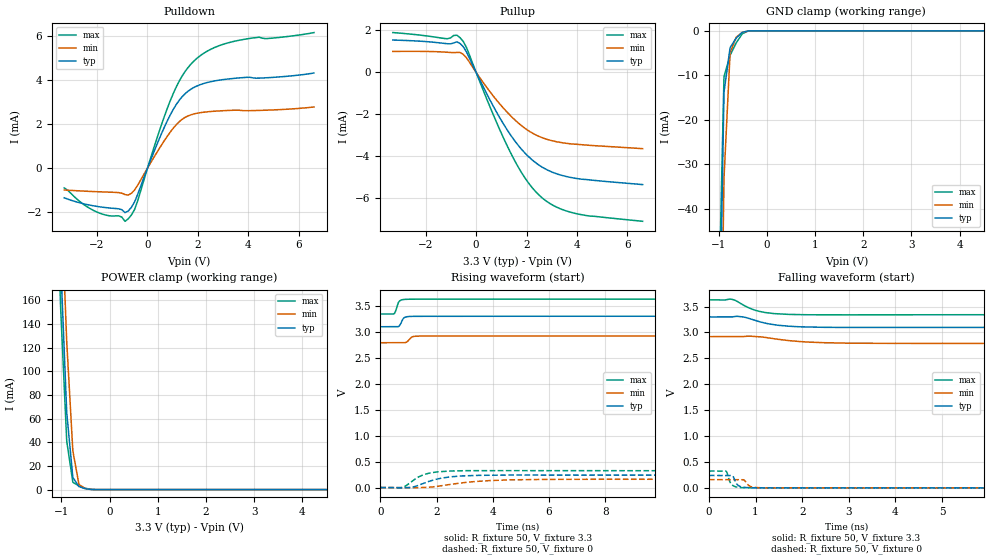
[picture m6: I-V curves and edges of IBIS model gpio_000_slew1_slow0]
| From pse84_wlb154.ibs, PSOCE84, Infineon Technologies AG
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[Model] gpio_000_slew1_slow0
Model_type I/O
Enable   Active-High
Vinl  =  0.99
Vinh  =  2.31
Vmeas =  1.65
Cref  =  15e-12
| Capacitance   typ   min   max
C_comp   1.09946e-12   1.086232e-12   1.114407e-12
| Variables   typ   min   max
[GND Clamp Reference]   0   0   0
[POWER Clamp Reference]   3.3   2.92   3.63
[Pulldown Reference]   0   0   0
[Pullup Reference]   3.3   2.92   3.63
[Temperature Range]   25   125   -40
[Voltage Range]   3.3   2.92   3.63
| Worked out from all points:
|   slope of the pulldown table from 0 to 0.495 V, typ, clamps not added: 352 ohm
|   slope of the pullup table from 0 to 0.495 V, typ, clamps not added: 415 ohm
|   GND clamp passes 1 mA (typ) near -0.57 V on its own axis
|   POWER clamp passes 1 mA (typ) near -0.52 V on its own axis
|   falling waveform, R_fixture 50, V_fixture 3.3: 20-80 % time 594ps typ, 820ps min, 464ps max; typ from 3.3 V to 3.1 V
|   falling waveform, R_fixture 50, V_fixture 0: 20-80 % time 91.4ps typ, 98.1ps min, 88.6ps max; typ from 0.239 V to 0 V
|   rising waveform, R_fixture 50, V_fixture 3.3: 20-80 % time 118ps typ, 140ps min, 107ps max; typ from 3.1 V to 3.3 V
|   rising waveform, R_fixture 50, V_fixture 0: 20-80 % time 912ps typ, 1.55ns min, 627ps max; typ from 0 V to 0.239 V
[GND Clamp]
| Voltage   I(typ)   I(min)   I(max)
-1.65V    -892.5mA   -911.9mA   -883.9mA
-1.015V   -92.32mA   -129.7mA   -71.28mA
-888.3mV  -13.83mA   -33.21mA   -10.31mA
-761.4mV  -3.792mA   -4.944mA   -5.509mA
-634.5mV  -1.622mA   -1.436mA   -2.707mA
-507.6mV  -326.2uA   -352.3uA   -651.6uA
-380.7mV  -13.48uA   -32.14uA   -19.55uA
-253.8mV  -189.4nA   -1.276uA   -466.7nA
6.6V      0A         0A         0A
[POWER Clamp]
| Voltage   I(typ)   I(min)   I(max)
-1.523V   838.1mA    872.9mA    823.9mA
-1.142V   346.5mA    405.1mA    310.5mA
-1.015V   193mA      257.4mA    153.9mA
-888.3mV  64.97mA    124.9mA    40.96mA
-761.4mV  10.28mA    32.7mA     6.184mA
-634.5mV  2.553mA    4.346mA    3.067mA
-507.6mV  805.9uA    960.7uA    1.159mA
-253.8mV  1.454uA    10.02uA    1.678uA
6.6V      0A         0A         0A
[Pulldown]
| Voltage   I(typ)   I(min)   I(max)
-3.3V     -1.344mA   -988.2uA   -894.2uA
-2.284V   -1.677mA   -1.054mA   -1.827mA
-1.142V   -1.844mA   -1.108mA   -2.163mA
-888.3mV  -2.016mA   -1.199mA   -2.411mA
-507.6mV  -1.525mA   -984.7uA   -1.869mA
455.2mV   1.299mA    868.4uA    1.635mA
1.024V    2.673mA    1.819mA    3.396mA
1.366V    3.234mA    2.212mA    4.169mA
1.821V    3.655mA    2.458mA    4.843mA
2.503V    3.928mA    2.575mA    5.397mA
3.425V    4.079mA    2.633mA    5.759mA
6.6V      4.324mA    2.781mA    6.16mA
[Pullup]
| Voltage   I(typ)   I(min)   I(max)
-3.3V     1.542mA    997.6uA    1.899mA
-1.142V   1.367mA    959.3uA    1.605mA
-761.4mV  1.457mA    951.8uA    1.773mA
-634.5mV  1.377mA    947.3uA    1.655mA
-380.7mV  976.2uA    696.2uA    1.185mA
682.8mV   -1.619mA   -1.133mA   -2.028mA
1.479V    -3.183mA   -2.206mA   -4.102mA
2.048V    -3.99mA    -2.766mA   -5.236mA
2.731V    -4.604mA   -3.17mA    -6.102mA
3.3V      -4.885mA   -3.339mA   -6.496mA
4.051V    -5.082mA   -3.443mA   -6.768mA
6.6V      -5.362mA   -3.644mA   -7.113mA
[Ramp]
dV/dt_r   0.143584/0.912412n  95.459m/1.55235n  0.194972/0.626948n
dV/dt_f   0.121179/0.594134n  77.9607m/0.820397n  0.172121/0.463712n
R_load = 50
[Falling Waveform]
R_fixture = 50
V_fixture = 3.3
V_fixture_min = 2.92
V_fixture_max = 3.63
| Time   V(typ)   V(min)   V(max)
0s        3.3V       2.92V      3.63V
506.7ps   3.301V     2.92V      3.638V
598.5ps   3.313V     2.92V      3.604V
727.5ps   3.301V     2.92V      3.535V
991.6ps   3.233V     2.922V     3.429V
1.21ns    3.18V      2.904V     3.385V
1.403ns   3.149V     2.878V     3.364V
1.887ns   3.113V     2.829V     3.346V
2.741ns   3.098V     2.798V     3.341V
800ns     3.098V     2.79V      3.343V
[Falling Waveform]
R_fixture = 50
V_fixture = 0
V_fixture_min = 0
V_fixture_max = 0
| Time   V(typ)   V(min)   V(max)
0s        239.3mV    159.1mV    325mV
367.6ps   239.2mV    159mV      320.9mV
468.4ps   239.3mV    159mV      87.18mV
517.8ps   221mV      159.1mV    42.82mV
589.1ps   84.64mV    159.2mV    16.49mV
745.8ps   10.57mV    154mV      2.516mV
857.1ps   3.295mV    43.44mV    1.058mV
949.8ps   1.519mV    12.37mV    758.9uV
1.62ns    307.6uV    296.1uV    276uV
800ns     26.22nV    728.5nV    16.41nV
[Rising Waveform]
R_fixture = 50
V_fixture = 3.3
V_fixture_min = 2.92
V_fixture_max = 3.63
| Time   V(typ)   V(min)   V(max)
0s        3.098V     2.79V      3.343V
486.3ps   3.098V     2.79V      3.348V
540.3ps   3.098V     2.79V      3.395V
650.8ps   3.104V     2.79V      3.572V
786.7ps   3.229V     2.79V      3.619V
901.5ps   3.285V     2.794V     3.626V
1.104ns   3.297V     2.893V     3.628V
1.198ns   3.298V     2.912V     3.629V
2.403ns   3.3V       2.919V     3.63V
800ns     3.3V       2.92V      3.63V
[Rising Waveform]
R_fixture = 50
V_fixture = 0
V_fixture_min = 0
V_fixture_max = 0
| Time   V(typ)   V(min)   V(max)
0s        26.29nV    727.8nV    16.58nV
779.6ps   -1.693mV   201.4uV    27.22uV
1.072ns   1.352mV    -997.5uV   99.81mV
1.353ns   42.96mV    -1.08mV    202.2mV
1.778ns   127.4mV    8.3mV      282.5mV
2.498ns   207mV      61.52mV    319.2mV
3.916ns   237.7mV    134.9mV    327mV
5.607ns   241mV      156.6mV    325.8mV
9.227ns   239.8mV    160.4mV    324.9mV
800ns     239.3mV    159.1mV    325mV
